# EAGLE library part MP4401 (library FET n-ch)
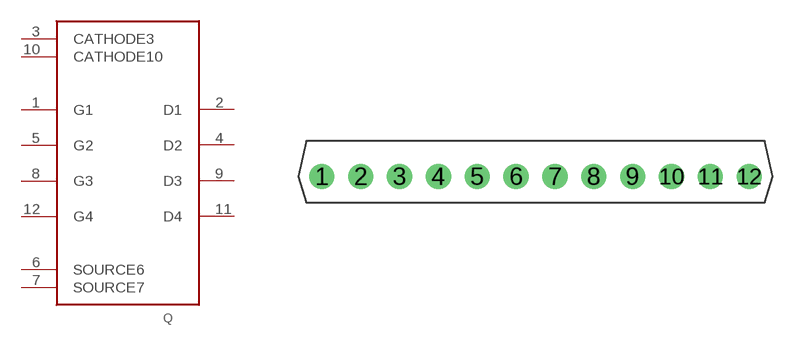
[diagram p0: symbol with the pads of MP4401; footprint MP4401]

Designator prefix Q

## MP4401  [MP4401]
1  G1
2  D1
3  CATHODE3
4  D2
5  G2
6  SOURCE6  pwr
7  SOURCE7  pwr
8  G3
9  D3
10  CATHODE10
11  D4
12  G4

## Footprint MP4401 (pad centres in mm)
MP4401 is a n ch FET, by TOSHIBA (follow data is from Akituki)秋月電子 ----------------------------------------------------- ■シングルインライン１２ピン ■モータードライブ・ソレノイドなどに最適！ ◆ＶＤＳＳ：１２０Ｖ ◆ＩＤ：３Ａ（ピーク１２Ａ）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
drill 1.1: 1 -13.97,0; 2 -11.43,0; 3 -8.89,0; 4 -6.35,0; 5 -3.81,0; 6 -1.27,0; 7 1.27,0; 8 3.81,0; 9 6.35,0; 10 8.89,0; 11 11.43,0; 12 13.97,0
